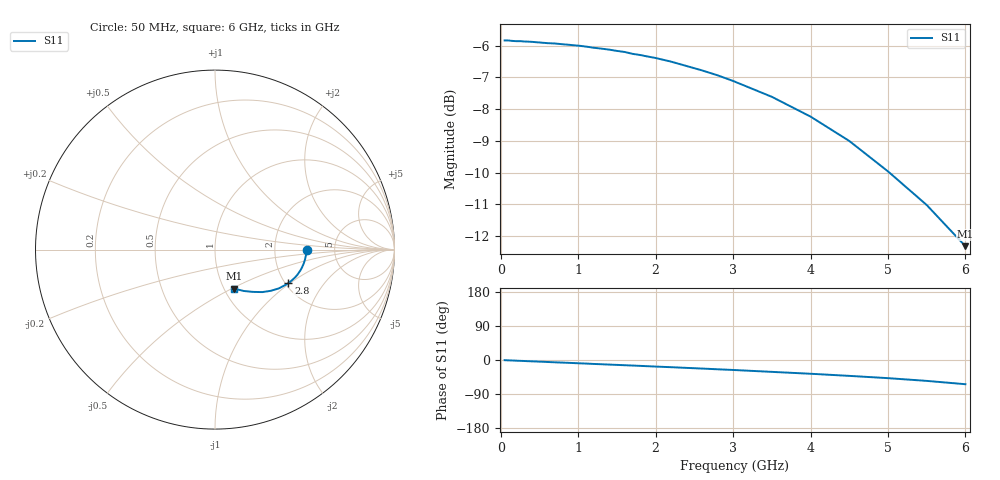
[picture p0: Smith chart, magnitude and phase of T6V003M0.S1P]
! SIEMENS Discrete & RF Semiconductors
! BAT62
! Si Schottky Diode in SOT143
! IF = 3 mA
! S-Parameters:  February  1997
# GHz  S  MA  R  50
!  f  S11
! GHz  MAG  ANG
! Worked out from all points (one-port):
!   34 points, 50 MHz to 6 GHz, reference 50 ohm
!   lowest |S11| = -12.3 dB at 6 GHz (marker M1), VSWR 1.64, Z = 55.7 - j25.7 ohm
!   |S11| at or under -10 dB: 5.017 GHz to end of sweep
!   S11 on the Smith chart (normalised r, x): 50 MHz: 3.09, -0.04; 2.8 GHz: 2.08, -0.97; 6 GHz: 1.11, -0.51
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0.05  0.5105 -0.5
0.1  0.5105 -0.9
0.15  0.5097 -1.3
0.2  0.5091 -1.8
0.3  0.5086 -2.6
0.4  0.508 -3.5
0.5  0.5068 -4.3
0.7  0.5049 -6.1
0.8  0.5035 -6.9
1.1  0.4993 -9.4
1.2  0.4971 -10.4
1.3  0.4956 -11.2
1.4  0.4938 -12.1
1.6  0.4896 -13.8
1.7  0.4864 -14.6
1.8  0.4842 -15.5
2  0.479 -17.3
2.2  0.4727 -19.0
2.4  0.4653 -20.8
2.6  0.4579 -22.6
2.8  0.4499 -24.5
3  0.4408 -26.3
3.5  0.4162 -31.3
4  0.3873 -36.3
4.5  0.3546 -41.9
5  0.3176 -47.9
5.5  0.2811 -55.1
6  0.2421 -63.9
